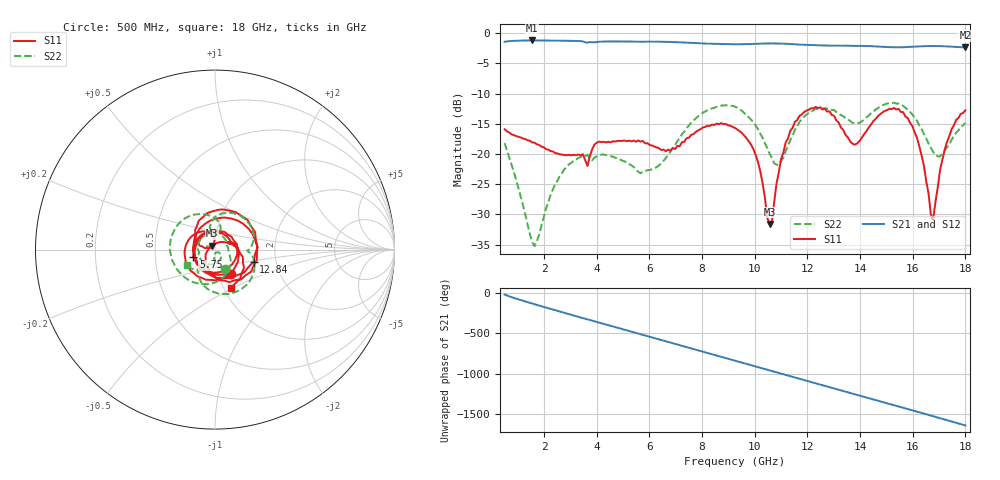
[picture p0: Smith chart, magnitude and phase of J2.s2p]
!Agilent Technologies,N5230C,MY49001096,A.09.42.15
!Agilent N5230C: A.09.42.15
!Date: Thursday, June 29, 2023 08:10:57
!Correction: S11(Full 2 Port(1,2))
!S21(Full 2 Port(1,2))
!S12(Full 2 Port(1,2))
!S22(Full 2 Port(1,2))
!S2P File: Measurements: S11, S21, S12, S22:
# Hz S  dB  R 50
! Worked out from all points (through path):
!   201 points, 500 MHz to 18 GHz, reference 50 ohm
!   highest |S21| = -1.20 dB at 1.55 GHz (marker M1); lowest = -2.4 dB at 18 GHz (marker M2)
!   group delay of S21, straight-line fit = 254 ps
!   lowest |S11| = -31.6 dB at 10.56 GHz (marker M3), VSWR 1.05, Z = 48.4 + j2.08 ohm
!   |S11| at or under -10 dB: start of sweep to end of sweep
!   |S22| runs from -35.3 to -11.5 dB; largest |S21 - S12| = 0.0013
!   S11 on the Smith chart (normalised r, x): 500 MHz: 1.14, -0.32; 5.75 GHz: 0.78, -0.07; 12.84 GHz: 1.53, -0.22; 18 GHz: 1.09, -0.48
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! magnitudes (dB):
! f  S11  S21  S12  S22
! 500 MHz  -15.9  -1.4  -1.4  -18.2
! 1.55 GHz  -18.1  -1.2  -1.2  -34.6
! 2.6 GHz  -20.1  -1.2  -1.2  -23.6
! 3.475 GHz  -20.1  -1.4  -1.4  -20.2
! 3.65 GHz  -22.0  -1.6  -1.6  -20.1
! 4.088 GHz  -18.0  -1.4  -1.4  -20.1
! 5.75 GHz  -17.9  -1.4  -1.4  -22.9
! 6.362 GHz  -19.1  -1.4  -1.4  -21.9
! 7.85 GHz  -16.1  -1.7  -1.7  -13.8
! 9.25 GHz  -15.7  -1.8  -1.8  -12.2
! 10.04 GHz  -20.2  -1.8  -1.8  -15.3
! 10.56 GHz  -31.6  -1.7  -1.7  -20.0
! 10.91 GHz  -23.1  -1.7  -1.7  -21.9
! 11.18 GHz  -18.1  -1.8  -1.8  -19.5
! 12.22 GHz  -12.4  -2.0  -2.0  -12.8
! 12.84 GHz  -12.9  -2.1  -2.1  -12.5
! 13.8 GHz  -18.5  -2.1  -2.1  -14.9
! 15.11 GHz  -12.5  -2.3  -2.3  -11.6
! 16.16 GHz  -17.3  -2.2  -2.2  -14.5
! 16.77 GHz  -30.9  -2.1  -2.1  -19.6
! 17.21 GHz  -19.3  -2.2  -2.2  -19.4
! 18 GHz  -12.8  -2.4  -2.4  -14.9
